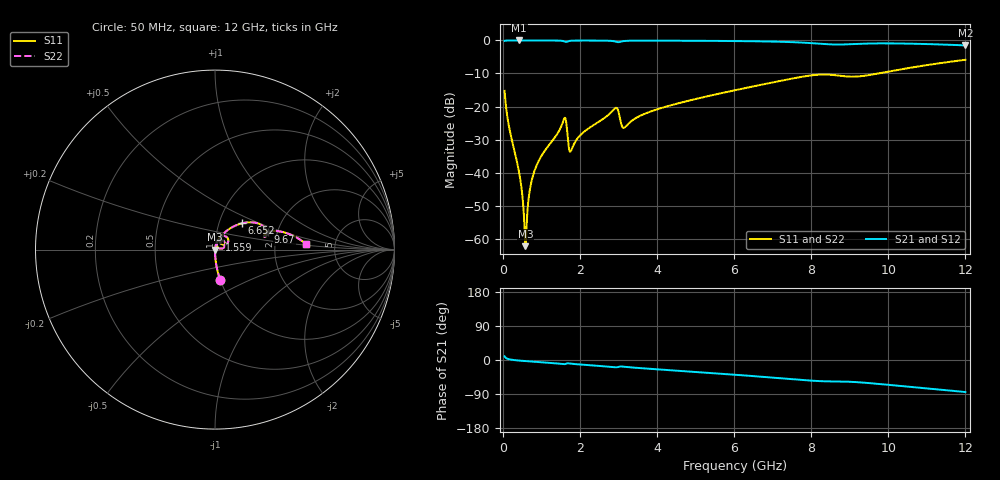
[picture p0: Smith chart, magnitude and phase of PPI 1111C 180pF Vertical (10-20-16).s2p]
# GHz S MA R 50
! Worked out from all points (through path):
!   1601 points, 50 MHz to 12 GHz, reference 50 ohm
!   highest |S21| = -0.01 dB at 430.9 MHz (marker M1); lowest = -1.5 dB at 12 GHz (marker M2)
!   group delay of S21, straight-line fit = 19.3 ps
!   lowest |S11| = -62.3 dB at 587.8 MHz (marker M3), VSWR 1.00, Z = 50.1 - j0.0202 ohm
!   |S11| at or under -10 dB: start of sweep to 9.742 GHz
!   |S22| runs from -62.3 to -5.9 dB; largest |S21 - S12| = 0
!   S11 on the Smith chart (normalised r, x): 50 MHz: 1.00, -0.35; 1.559 GHz: 1.05, +0.11; 6.652 GHz: 1.29, +0.39; 9.67 GHz: 1.78, +0.38; 12 GHz: 3.06, +0.25
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0.05  0.1725 -80.2  0.9847 9.7  0.9847 9.7  0.1725 -80.2
0.1769688  0.04539 -87.7  0.9985 1.7  0.9985 1.7  0.04539 -87.7
0.4309062  0.0097 -87.7  0.9993 -1.6  0.9993 -1.6  0.0097 -87.7
0.4906563  0.005697 -85.1  0.9993 -2.1  0.9993 -2.1  0.005697 -85.1
0.5504062  0.002278 -73.9  0.9992 -2.6  0.9992 -2.6  0.002278 -73.9
0.58775  0.0007699 -15.2  0.9992 -2.9  0.9992 -2.9  0.0007699 -15.2
0.6325625  0.002221 66.3  0.9992 -3.2  0.9992 -3.2  0.002221 66.3
0.7296563  0.006597 78.8  0.9991 -3.9  0.9991 -3.9  0.006597 78.8
0.8491562  0.01161 80.6  0.999 -4.8  0.999 -4.8  0.01161 80.6
1.558688  0.05762 63.3  0.9826 -10.8  0.9826 -10.8  0.05762 63.3
1.625906  0.06644 33.3  0.9509 -10.6  0.9509 -10.6  0.06644 33.3
1.760344  0.02086 45.6  0.9878 -9.6  0.9878 -9.6  0.02086 45.6
2.044156  0.03833 73.1  0.996 -12.2  0.996 -12.2  0.03833 73.1
2.918  0.09472 51.1  0.9641 -19.3  0.9641 -19.3  0.09472 51.1
3.149531  0.04765 48.0  0.9793 -17.8  0.9793 -17.8  0.04765 48.0
4.038312  0.09188 63.2  0.9923 -24.8  0.9923 -24.8  0.09188 63.2
6.025  0.1764 49.5  0.9789 -38.9  0.9789 -38.9  0.1764 49.5
6.652375  0.2103 44.1  0.9693 -43.7  0.9693 -43.7  0.2103 44.1
8.019156  0.2966 26.4  0.9094 -54.6  0.9094 -54.6  0.2966 26.4
9.66975  0.3107 18.2  0.9009 -62.4  0.9009 -62.4  0.3107 18.2
10.01331  0.3383 17.7  0.9021 -65.6  0.9021 -65.6  0.3383 17.7
12  0.5098 3.4  0.8411 -84.5  0.8411 -84.5  0.5098 3.4
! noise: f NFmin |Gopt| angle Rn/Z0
0.05  0.0003684  0.8648  0.3511  0.0005851
1.372  0.005633  0.7703  6.639  0.004981
2.701  0.01225  0.7913  13.03  0.01195
4.031  0.01114  0.6826  19.09  0.006623
5.36  0.01375  0.6673  24.98  0.007578
6.682  0.02251  0.7411  31.12  0.0162
8.012  0.05859  0.8747  37.37  0.09063
9.341  0.07588  0.8895  43.06  0.1294
10.67  0.05154  0.8262  48.16  0.05207
12  0.0458  0.7919  52.9  0.03652
